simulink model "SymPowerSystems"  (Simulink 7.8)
settings: Solver=ode45  StartTime=0.0  StopTime=0.2  RelTol=1e-3
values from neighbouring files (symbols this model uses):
  C = 3*C    (= 0.0039788735773)    [parametri.m]
  Lm = (9.3e-3)/W    (= 2.96028194151e-05)    [parametri.m]
  Rm = 1.6e-3    (= 0.0016)    [parametri.m]
libraries: powerlib x8

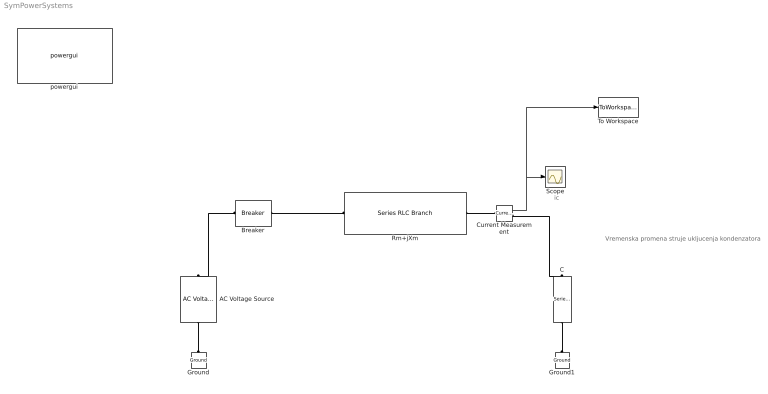
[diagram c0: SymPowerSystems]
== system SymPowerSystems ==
  note: ic
  note: Vremenska promena struje ukljucenja kondenzatora
  AC Voltage Source : powerlib/Electrical Sources/AC Voltage Source  Amplitude=230*sqrt(2)  Phase=90  Frequency=50  SampleTime=0  Measurements=None
  Breaker : powerlib/Elements/Breaker  BreakerResistance=0  InitialState=0  SnubberResistance=inf  SnubberCapacitance=inf  SwitchingTimes="[ 0/50  1000/50 ]"  External=off  Measurements=None  MoreParameters=off  NoBreakLoop=off
  C : powerlib/Elements/Series RLC Branch  LConnTagsString=__new0  RConnTagsString=__new0  BranchType=C  Resistance=1  Inductance=1e-3  SetiL0=off  InitialCurrent=0  Capacitance=C  Setx0=on  InitialVoltage=-230*sqrt(2)  Measurements=None
  Current Measurement : powerlib/Measurements/Current Measurement  PhasorSimulation=off  OutputType=Complex  PSBequivalent=0
  Ground : powerlib/Elements/Ground  LConnTagsString=a
  Ground1 : powerlib/Elements/Ground  LConnTagsString=a
  Rm+jXm : powerlib/Elements/Series RLC Branch  LConnTagsString=__new0  RConnTagsString=__new0  BranchType=RL  Resistance=Rm  Inductance=Lm  SetiL0=off  InitialCurrent=0  Capacitance=1e-6  Setx0=off  InitialVoltage=0  Measurements=None
  Scope : Scope
  To Workspace : ToWorkspace  VariableName=struja_ic_1  SampleTime=-1  SaveFormat=Structure With Time
  powergui : powerlib/powergui  Priority=1  SimulationMode=Continuous  SolverType=Tustin  SampleTime=50e-6  frequency=60  SPID=on  DisableSnubberDevices=on  DisableRonSwitches=on  DisableVfSwitches=on  SwTol=0  Interpol=off  DisplayEquations=on  FunctionMessages=off  frequencyindice=50  Pbase=100e6  ErrMax=1e-4  Iterations=50  UnitsV=kV  UnitsW=MW  echomessages=off  HookPort=off  EnableUseOfTLC=off  x0status=blocks  RestoreLinks=warning  ResistiveCurrentMeasurement=off  Ylog=off  Xlog=on  ShowGrid=off  save=off  variable=ZData  ZoomFFT=off  StartTime=0.0  cycles=1  DisplayStyle=1  FreqAxis=off  MaxFrequency=1000  frequencyindicesteady=1  RmsSteady=2  display=off  methode=off
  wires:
  Current Measurement/1 -> Scope/1, To Workspace/1
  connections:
  C/RConn1 -- Ground1/LConn1
  AC Voltage Source/LConn1 -- Ground/LConn1
  Current Measurement/LConn1 -- Rm+jXm/RConn1
  Current Measurement/RConn1 -- C/LConn1
  Breaker/RConn1 -- Rm+jXm/LConn1
  Breaker/LConn1 -- AC Voltage Source/RConn1
